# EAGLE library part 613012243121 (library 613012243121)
WURTH ELEKTRONIK - 613012243121 - CONNECTOR, RCPT, 12POS, 2ROW, 2.54MM Source: Datasheet
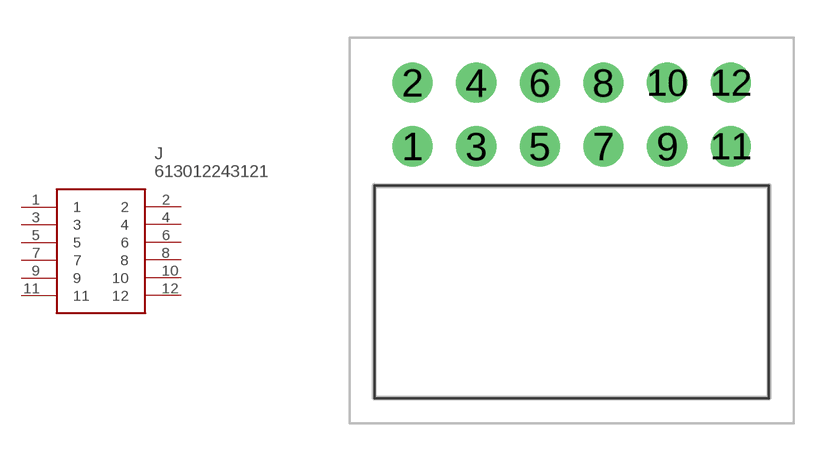
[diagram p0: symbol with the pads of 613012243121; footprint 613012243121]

Designator prefix J

## 613012243121 (Description: WURTH ELEKTRONIK - 613012243121 - CONNECTOR, RCPT, 12POS, 2ROW, 2.54MM; Height: 5.23mm; Manufacturer_Name: Wurth Elektronik; Manufacturer_Part_Number: 613012243121; Mouser_Part_Number: 710-613012243121; Mouser_Price-Stock: https://www.mouser.co.uk/ProductDetail/Wurth-Elektronik/613012243121?qs=iLbezkQI%252Bsgb444HYkTruQ%3D%3D)  [613012243121]
1  1
2  2
3  3
4  4
5  5
6  6
7  7
8  8
9  9
10  10
11  11
12  12

## Footprint 613012243121 (pad centres in mm)
613012243121-1
drill 1.07 pad 1.605: 1 0,0; 2 0,2.54; 3 2.54,0; 4 2.54,2.54; 5 5.08,0; 6 5.08,2.54; 7 7.62,0; 8 7.62,2.54; 9 10.16,0; 10 10.16,2.54; 11 12.7,0; 12 12.7,2.54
